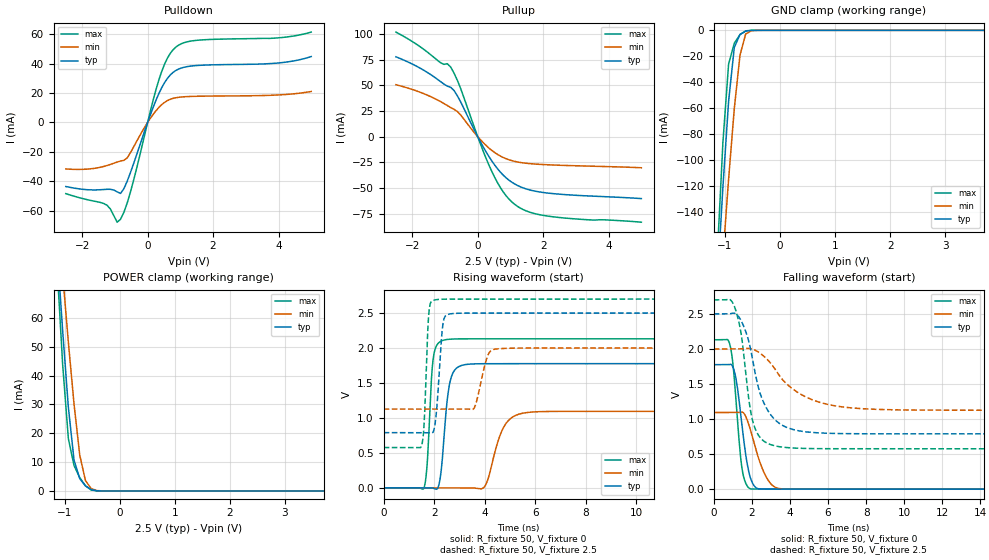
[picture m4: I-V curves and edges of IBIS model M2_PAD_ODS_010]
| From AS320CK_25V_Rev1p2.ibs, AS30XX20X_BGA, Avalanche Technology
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[Model] M2_PAD_ODS_010
Model_type I/O
Enable   Active-High
Vinl  =  0.7
Vinh  =  1.8
Vmeas =  1.25
Cref  =  30e-12
| Capacitance  typ   min   max
C_comp   1.568193e-12   1.472592e-12   1.715469e-12
| Variables   typ   min   max
[GND Clamp Reference]   0   0   0
[POWER Clamp Reference]   2.5   2   2.7
[Pulldown Reference]   0   0   0
[Pullup Reference]   2.5   2   2.7
[Temperature Range]   25   125   -40
[Voltage Range]   2.5   2   2.7
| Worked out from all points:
|   slope of the pulldown table from 0 to 0.375 V, typ, clamps not added: 17.8 ohm
|   slope of the pullup table from 0 to 0.375 V, typ, clamps not added: 18 ohm
|   GND clamp passes 1 mA (typ) near -0.64 V on its own axis
|   POWER clamp passes 1 mA (typ) near -0.56 V on its own axis
|   falling waveform, R_fixture 50, V_fixture 0: 20-80 % time 505ps typ, 778ps min, 385ps max; typ from 1.78 V to 0 V
|   falling waveform, R_fixture 50, V_fixture 2.5: 20-80 % time 1.03ns typ, 2.06ns min, 615ps max; typ from 2.5 V to 0.789 V
|   rising waveform, R_fixture 50, V_fixture 0: 20-80 % time 269ps typ, 559ps min, 183ps max; typ from 0 V to 1.78 V
|   rising waveform, R_fixture 50, V_fixture 2.5: 20-80 % time 193ps typ, 337ps min, 136ps max; typ from 0.789 V to 2.5 V
[GND Clamp]
| Voltage   I(typ)   I(min)   I(max)
-2.5V     -1.297A    -1.146A    -1.538A
-1.138V   -195.9mA   -238.3mA   -175.2mA
-1.034V   -121.2mA   -175.1mA   -86.57mA
-931mV    -54.79mA   -114.9mA   -26.01mA
-827.6mV  -13.15mA   -60.41mA   -9.967mA
-724.1mV  -3.205mA   -19.15mA   -3.28mA
-620.7mV  -615.3uA   -2.798mA   -407.6uA
-517.2mV  -34.39uA   -319.4uA   -6.513uA
-413.8mV  -821.3nA   -24.43uA   -50.96nA
5V        0A         0A         0A
[POWER Clamp]
| Voltage   I(typ)   I(min)   I(max)
-2.5V     511mA      454.9mA    606.6mA
-1.138V   84.76mA    99.9mA     78.64mA
-1.034V   55.67mA    75.27mA    43.94mA
-931mV    29.07mA    51.7mA     18.16mA
-827.6mV  10.68mA    30.08mA    8.788mA
-724.1mV  4.238mA    12.45mA    4.618mA
-620.7mV  1.771mA    3.587mA    1.776mA
-517.2mV  465uA      837.9uA    329.7uA
-413.8mV  47.65uA    120.2uA    11.19uA
-310.3mV  1.515uA    11.72uA    116.8nA
5V        0A         0A         0A
[Pulldown]
| Voltage   I(typ)   I(min)   I(max)
-2.5V     -43.54mA   -31.62mA   -48.38mA
-1.345V   -45.58mA   -29.95mA   -55.04mA
-1.138V   -45.44mA   -28.55mA   -58.81mA
-931mV    -47.17mA   -26.91mA   -67.8mA
-827.6mV  -48.24mA   -26.21mA   -65.83mA
-517.2mV  -33.61mA   -20.26mA   -46.69mA
344.8mV   19.68mA    10.22mA    29mA
603.4mV   29.91mA    14.84mA    43.66mA
948.3mV   36.32mA    17.11mA    52.56mA
1.638V    38.89mA    17.86mA    56.1mA
3.99V     40.44mA    18.69mA    57.52mA
5V        44.82mA    21.06mA    61.44mA
[Pullup]
| Voltage   I(typ)   I(min)   I(max)
-2.5V     77.66mA    50.55mA    101.7mA
-1.552V   62.71mA    40.56mA    82.54mA
-1.138V   53.61mA    34.15mA    71.93mA
-827.6mV  48.08mA    28.39mA    67.76mA
-517.2mV  33.57mA    20.94mA    46.41mA
86.21mV   -5.185mA   -3.042mA   -7.343mA
431mV     -23.58mA   -13.31mA   -33.77mA
775.9mV   -37.21mA   -20.13mA   -53.46mA
1.121V    -45.74mA   -23.87mA   -65.48mA
1.552V    -51.37mA   -26mA      -72.89mA
2.155V    -54.78mA   -27.26mA   -77.18mA
5V        -60.09mA   -30.14mA   -83.02mA
[Ramp]
dV/dt_r   1.06541/0.26881n  0.65595/0.55939n  1.27868/0.183118n
dV/dt_f   1.02665/1.03344n  0.524479/2.05985n  1.27424/0.615015n
R_load = 50
[Falling Waveform]
R_fixture = 50
V_fixture = 0
V_fixture_min = 0
V_fixture_max = 0
| Time   V(typ)   V(min)   V(max)
0s        1.776V     1.093V     2.131V
853.4ps   1.78V      1.094V     2.054V
997.5ps   1.746V     1.094V     1.808V
1.167ns   1.575V     1.094V     1.266V
1.457ns   968.2mV    1.099V     345.3mV
1.616ns   613.4mV    1.069V     129.8mV
1.903ns   181mV      866.8mV    7.495mV
2.701ns   2.004mV    201.7mV    764.5uV
3.407ns   915.4uV    9.526mV    418uV
21.88ns   -194.7nV   403.6pV    -423.4nV
[Falling Waveform]
R_fixture = 50
V_fixture = 2.5
V_fixture_min = 2
V_fixture_max = 2.7
| Time   V(typ)   V(min)   V(max)
0s        2.5V       2V         2.7V
1.078ns   2.51V      2V         2.613V
1.422ns   2.413V     2.001V     2.242V
1.827ns   2.119V     2.008V     1.309V
2.055ns   1.828V     1.995V     959.7mV
2.453ns   1.35V      1.936V     730mV
2.999ns   1.057V     1.793V     633.9mV
4.478ns   831.9mV    1.369V     583.4mV
6.697ns   792.9mV    1.175V     576.6mV
21.88ns   788.9mV    1.126V     576.3mV
[Rising Waveform]
R_fixture = 50
V_fixture = 0
V_fixture_min = 0
V_fixture_max = 0
| Time   V(typ)   V(min)   V(max)
0s        2.114nV    46.37nV    1.824nV
1.601ns   -420uV     -435.4uV   523.8uV
1.97ns    -7.665mV   -535.7uV   1.865V
2.378ns   659.2mV    -646.7uV   2.113V
2.653ns   1.55V      -721.3uV   2.127V
3.242ns   1.763V     -881.5uV   2.131V
4.009ns   1.775V     21.73mV    2.131V
4.727ns   1.776V     847.2mV    2.131V
5.515ns   1.776V     1.067V     2.131V
21.88ns   1.776V     1.093V     2.131V
[Rising Waveform]
R_fixture = 50
V_fixture = 2.5
V_fixture_min = 2
V_fixture_max = 2.7
| Time   V(typ)   V(min)   V(max)
0s        788.9mV    1.126V     576.3mV
1.497ns   788.5mV    1.126V     597.7mV
1.602ns   788.5mV    1.126V     906.9mV
1.792ns   788.5mV    1.126V     2.506V
2.019ns   873.8mV    1.126V     2.687V
2.333ns   2.298V     1.127V     2.698V
2.591ns   2.485V     1.127V     2.699V
3.564ns   2.499V     1.13V      2.699V
4.436ns   2.499V     1.985V     2.699V
21.88ns   2.5V       2V         2.7V
